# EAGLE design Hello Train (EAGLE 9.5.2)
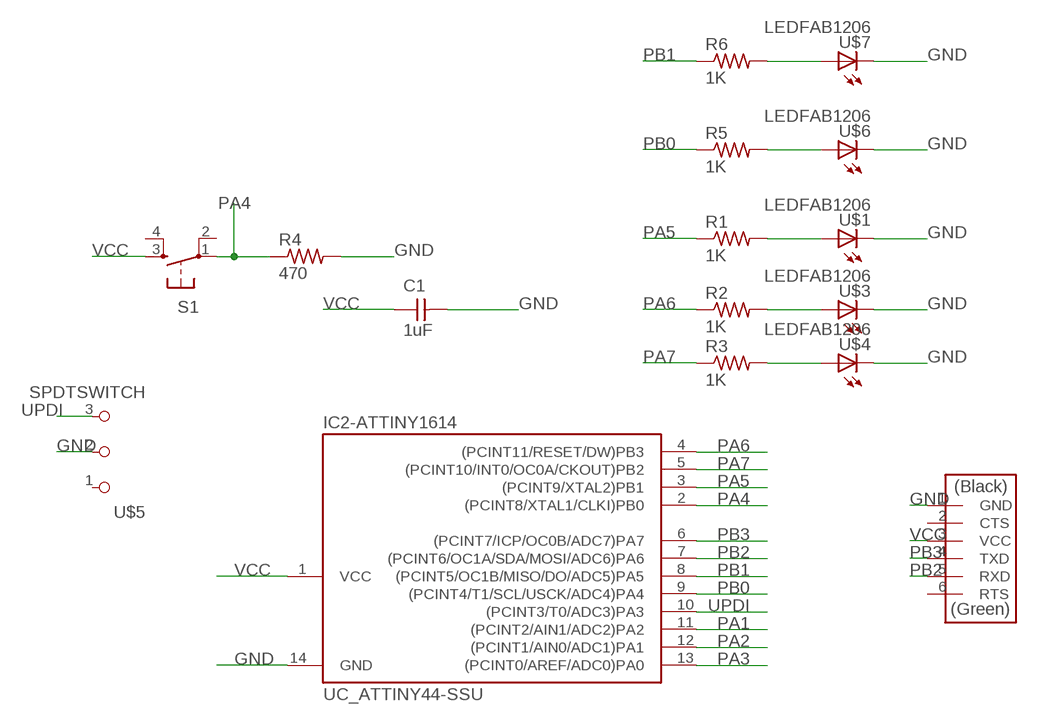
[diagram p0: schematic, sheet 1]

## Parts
C1  1uF  CAP_UNPOLARIZEDFAB  [C1206FAB]
IC2-ATTINY1614  UC_ATTINY44-SSU  [SOIC14]
R1  1K  R1206FAB  [R1206FAB]
R2  1K  R1206FAB  [R1206FAB]
R3  1K  R1206FAB  [R1206FAB]
R4  470  RES-US1206FAB  [R1206FAB]
R5  1K  R1206FAB  [R1206FAB]
R6  1K  R1206FAB  [R1206FAB]
S1  SW_SWITCH_TACTILE_6MM6MM_SWITCH  [6MM_SWITCH]
U$1  LEDFAB1206  [LED1206FAB]
U$2  CONN_06_FTDI-SMD-HEADER  [1X06SMD]
U$3  LEDFAB1206  [LED1206FAB]
U$4  LEDFAB1206  [LED1206FAB]
U$5  SPDTSWITCH  [SPDTSWITCH]
U$6  LEDFAB1206  [LED1206FAB]
U$7  LEDFAB1206  [LED1206FAB]

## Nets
GND: C1.2 IC2-ATTINY1614.14(GND) R4.2 U$1.2(C) U$2.1(GND) U$3.2(C) U$4.2(C) U$5.2 U$6.2(C) U$7.2(C)
N$1: R2.2 U$3.1(A)
N$2: R5.2 U$6.1(A)
N$3: R3.2 U$4.1(A)
N$4: R6.2 U$7.1(A)
N$7: R1.2 U$1.1(A)
PA1: IC2-ATTINY1614.11((PCINT2/AIN1/ADC2)PA2)
PA2: IC2-ATTINY1614.12((PCINT1/AIN0/ADC1)PA1)
PA3: IC2-ATTINY1614.13((PCINT0/AREF/ADC0)PA0)
PA4: IC2-ATTINY1614.2((PCINT8/XTAL1/CLKI)PB0) R4.1 S1.1(P)
PA5: IC2-ATTINY1614.3((PCINT9/XTAL2)PB1) R1.1
PA6: IC2-ATTINY1614.4((PCINT11/RESET/DW)PB3) R2.1
PA7: IC2-ATTINY1614.5((PCINT10/INT0/OC0A/CKOUT)PB2) R3.1
PB0: IC2-ATTINY1614.9((PCINT4/T1/SCL/USCK/ADC4)PA4) R5.1
PB1: IC2-ATTINY1614.8((PCINT5/OC1B/MISO/DO/ADC5)PA5) R6.1
PB2: IC2-ATTINY1614.7((PCINT6/OC1A/SDA/MOSI/ADC6)PA6) U$2.5(RXD)
PB3: IC2-ATTINY1614.6((PCINT7/ICP/OC0B/ADC7)PA7) U$2.4(TXD)
UPDI: IC2-ATTINY1614.10((PCINT3/T0/ADC3)PA3) U$5.3
VCC [New Class]: C1.1 IC2-ATTINY1614.1(VCC) S1.3(S) U$2.3(VCC)
Unconnected: S1.2(P1) S1.4(S1) U$2.2(CTS) U$2.6(RTS) U$5.1

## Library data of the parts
C1 = fab:CAP_UNPOLARIZED
IC2-ATTINY1614 = fab:UC_ATTINY44
R1-R3 R5 R6 = fab:R: Resistor (US Symbol)
R4 = fab:RES-US: Resistor (US Symbol)
S1 = fab:SW_SWITCH_TACTILE_6MM: OMRON SWITCH
U$1 U$3 U$4 U$6 U$7 = fab:LED: LED
U$2 = fab:CONN_06_FTDI-SMD-HEADER
U$5 = fab:SPDTSWITCH

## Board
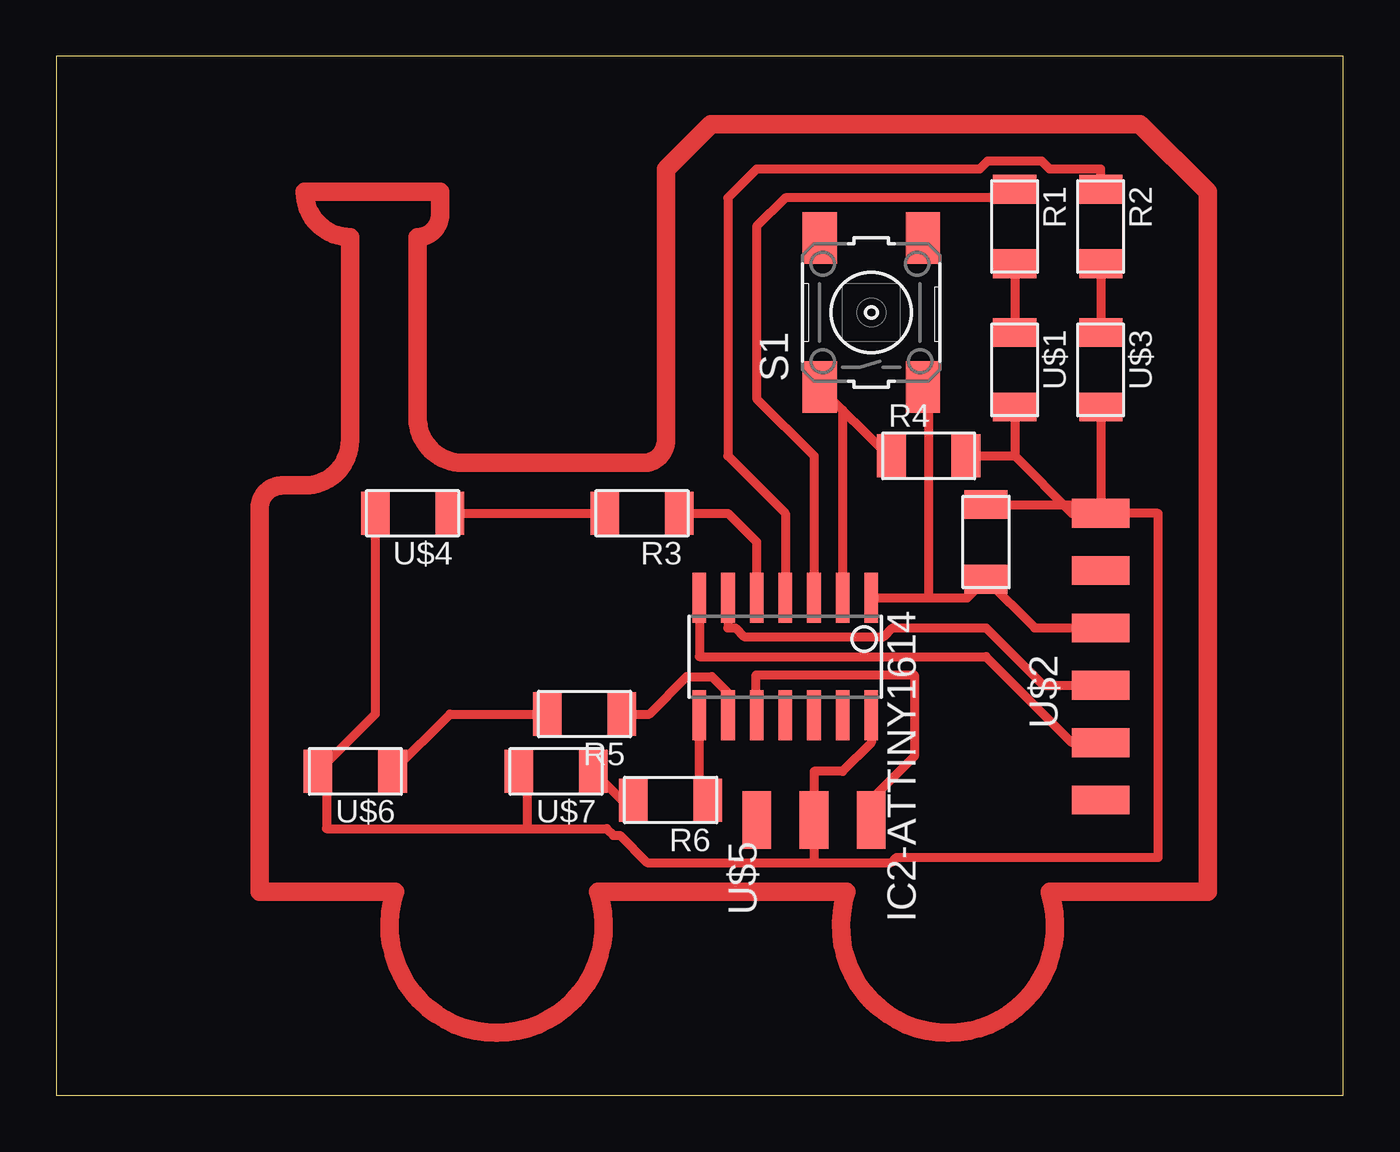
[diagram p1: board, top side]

Size 57 x 46 mm. Coordinates in mm from the lower left corner, seen from the top.
Outline: 0,0 57,0 57,46 0,46 0,0
Copper layers (1*16): Top 0.035mm / dielectric 1.5mm / Bottom 0.035mm
Design rules "default *": minimum track width 16mil, minimum drill 0.35mm, track to track 16mil, track to pad 16mil, pad to pad 16mil, via to via 16mil, smd to smd 16mil, copper to edge 40mil, drill to drill 6mil, minimum pad ring 10mil, minimum via ring 8mil, stop-mask expansion 4mil, vias tented up to drill 0mil, thermal gap 10mil

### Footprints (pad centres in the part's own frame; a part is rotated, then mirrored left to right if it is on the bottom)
C1206FAB = smd 1.27 x 1.905: 1 -1.651,0; 2 1.651,0
SOIC14 = smd 0.61 x 2.21: 1 -3.81,-2.603; 2 -2.54,-2.603; 3 -1.27,-2.603; 4 0,-2.603; 5 1.27,-2.603; 6 2.54,-2.603; 7 3.81,-2.603; 8 3.81,2.603; 9 2.54,2.603; 10 1.27,2.603; 11 0,2.603; 12 -1.27,2.603; 13 -2.54,2.603; 14 -3.81,2.603
R1206FAB = smd 1.27 x 1.905: 1 -1.651,0; 2 1.651,0
6MM_SWITCH = smd 2.286 x 1.524: 1 -3.302,2.286; 2 3.302,2.286; 3 -3.302,-2.286; 4 3.302,-2.286
LED1206FAB = smd 1.27 x 1.905: 1 -1.651,0; 2 1.651,0
1X06SMD = smd 2.54 x 1.27: 1 0,6.35; 2 0,3.81; 3 0,1.27; 4 0,-1.27; 5 0,-3.81; 6 0,-6.35
SPDTSWITCH = smd 2.54 x 1.27: 1 0.38,2.54; 2 0.38,0; 3 0.38,-2.54

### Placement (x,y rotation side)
C1  41.18,24.5 90 top
IC2-ATTINY1614  32.29,19.42 180 top
R1  42.45,38.47 270 top
R2  46.26,38.47 270 top
R3  25.94,25.77 180 top
R4  38.64,28.31 0 top
R5  23.4,16.88 180 top
R6  27.21,13.07 180 top
S1  36.1,34.66 90 top
U$1  42.45,32.12 270 top
U$2  46.26,19.42 0 top
U$3  46.26,32.12 270 top
U$4  15.78,25.77 180 top
U$5  33.56,11.8 90 top
U$6  13.24,14.34 180 top
U$7  22.13,14.34 180 top

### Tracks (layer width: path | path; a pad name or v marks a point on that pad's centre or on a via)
GND
  Top 0.406: IC2-ATTINY1614.14 36.1,15.61 34.83,14.34 33.56,14.34 U$5.2 33.56,10.3 | U$2.1 48.8,25.77 48.8,10.53 37.22,10.53 36.99,10.3 33.56,10.3 | 42.07,30.85 U$1.2 42.45,28.31 | C1.2 45.88,26.15 U$2.1 | U$3.2 U$2.1 | 42.45,28.31 44.99,25.77 U$2.1 | R4.2 42.45,28.31 | U$4.2 14.13,16.88 U$6.2 11.97,13.96 11.97,11.8 20.86,11.8 | 33.56,10.3 26.17,10.3 24.96,11.51 24.67,11.51 24.38,11.8 20.86,11.8 | U$7.2 20.86,13.96 20.86,11.8
N$1
  Top 0.406: R2.2 U$3.1
N$2
  Top 0.406: U$6.1 17.43,16.88 R5.2
N$3
  Top 0.406: U$4.1 R3.2
N$4
  Top 0.406: U$7.1 25.05,13.07 R6.2
N$6
  Top 0.813: 24,9 arc-217 15,9 9,9 9,26 arc-90 10,27 11,27 arc90 13,29 13,38 arc-90 11,40 17,40 17,39 arc-90 16,38 16,30 arc90 18,28 26,28 arc90 27,29 27,41 29,43 48,43 51,40 51,9 44,9 arc-217 35,9 24,9
N$7
  Top 0.406: R1.2 U$1.1
PA4
  Top 0.406: IC2-ATTINY1614.2 34.83,30.34 S1.1 36.86,28.31 R4.1
PA5
  Top 0.406: R1.1 42.07,39.74 32.29,39.74 31.02,38.47 31.02,30.85 33.56,28.31 IC2-ATTINY1614.3
PA6
  Top 0.406: R2.1 46.26,41.01 44.01,41.01 43.66,41.37 41.24,41.37 40.89,41.01 31.02,41.01 29.75,39.74 29.75,28.31 32.29,25.77 IC2-ATTINY1614.4
PA7
  Top 0.406: R3.1 29.75,25.77 31.02,24.5 IC2-ATTINY1614.5
PB0
  Top 0.406: R5.1 26.27,16.88 27.92,18.53 29.04,18.53 29.75,17.82 IC2-ATTINY1614.9
PB1
  Top 0.406: R6.1 28.48,13.45 IC2-ATTINY1614.8
PB2
  Top 0.406: IC2-ATTINY1614.7 28.48,19.42 41.18,19.42 44.99,15.61 U$2.5
PB3
  Top 0.406: IC2-ATTINY1614.6 29.75,20.69 30.08,20.69 30.46,20.31 36.66,20.31 37.04,20.69 41.18,20.69 43.72,18.15 U$2.4
UPDI
  Top 0.406: IC2-ATTINY1614.10 31,16.84 31,18.61 38,18.61 38,15 36,13 36,12.28 U$5.3
VCC
  Top 0.406: IC2-ATTINY1614.1 38.64,22.02 | 38.64,22.02 40.36,22.02 C1.1 43.34,20.69 U$2.3 | S1.3 38.64,31.1 38.64,22.02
